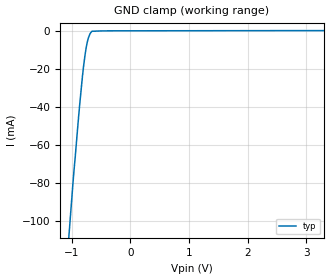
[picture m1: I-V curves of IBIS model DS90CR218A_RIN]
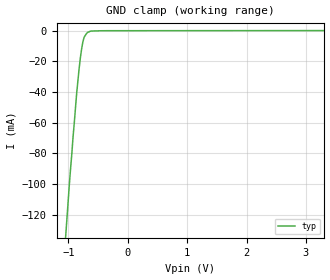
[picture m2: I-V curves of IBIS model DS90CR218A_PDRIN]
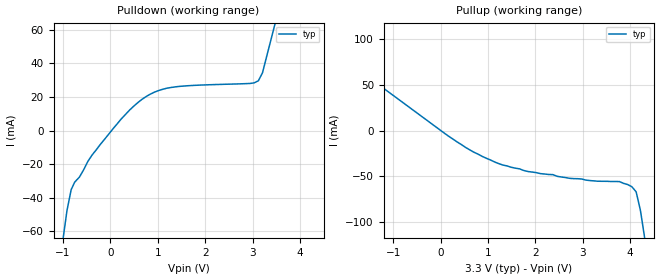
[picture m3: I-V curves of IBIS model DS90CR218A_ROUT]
|   National Semiconductor Corporation
|   Interface Products Group
|   IBIS Model of DS90CR218AMTD
|   High Speed Link Receiver
|   48L TSSOP
[IBIS Ver]   2.1
[Comment char]  |_char
[File name]   90cr218a.ibs
[File Rev]   1.3
[Date]   7/27/00
[Source]   File originated at National Semiconductor Corporation.
   Interface Group/Analog Division. All data based on
   Empirical Measurements(Bench).
[Notes]   File created by DT.
   Revision 1.0: The original model.
   Revision 1.1: Corrected driver output pulldown
   and pullup.
   Revision 1.2: Corrected ground and power clamp data.
   Revision 1.3: Changed Vih/Vil of LVDS Input to 100mV
   Deleted V/T data because it was wrong.
[Disclaimer]
(C) Copyright National Semiconductor Corporation 2000
   All rights reserved
   National Semiconductor Corporation hereby grants
the user of this IBIS model a non-exclusive, nontransferable
license to use this IBIS model under the following terms.
Before using this IBIS model, the user should read this
license.  If the user does not accept these terms, the
IBIS model should be returned to National within 30 days.
   The user is granted this license only to use the
IBIS model and is not granted rights to sell, load, rent,
lease or license the IBIS model in whole or in part, or in
modified form to anyone other than user. User may modify
the IBIS model to suit its specific applications but rights
to derivative works and such modifications shall belong to
National.
   This IBIS model is provided on an "AS IS" basis and
National makes absolutely no warranty with respect to the
information contained herein. NATIONAL DISCLAIMS AND CUSTOMER
WAIVES ALL WARRANTIES, EXPRESS OR IMPLIED, INCLUDING
WARRANTIES OF MERCHANTABILITY OR FITNESS FOR A PARTICULAR
PURPOSE. The entire risk as to quality and performance is
with the Customer. ACCORDINGLY, IN NO EVENT SHALL THE
COMPANY BE LIABLE FOR ANY DAMAGES, WHETHER IN CONTRACT OR
TORT,INCLUDING ANY LOST PROFITS OR OTHER INCIDENTAL,
CONSEQUENTIAL, EXEMPLARY, OR PUNITIVE DAMAGES ARISING OUT
OF THE USE OR APPLICATION OF THE IBIS model provided in
this package. Further, National reserves the right to make
changes without notice to any product herein to improve
reliability, function, or design. National does not convey
any license under patent rights or any other intellectual
property rights, including those of third parties.
   National is not obligated to provide maintenance or support
for the licensed IBIS model.
Contact National at ATTN:INTERFACE APPLICATIONS/IBIS MODELS.
2900 Semiconductor Drive, M/S A2595, Santa Clara, CA 95052-8090
[Copyright]   Copyright 2000, National Semiconductor, All Rights Reserved
[Component]   DS90CR218AMTD
[Manufacturer]  National Semiconductor Corp
[Package]
|   typ   min   max
R_pkg   97.97m   NA   NA
L_pkg   3.000nH   NA   NA
C_pkg   0.2108pF   NA   NA
[Pin]   signal_name   model_name   R_pin   L_pin   C_pin
1   RxOUT17   DS90CR218A_ROUT   68.8m  2.270n  0.3587p
2   RxOUT18   DS90CR218A_ROUT   65.4m  2.200n  0.3414p
3   GND   GND   133.7m  3.880n  0.3183p
4   RxOUT19   DS90CR218A_ROUT   121.7m  3.590n  0.2610p
5   RxOUT20   DS90CR218A_ROUT   120.6m  3.510n  0.2205p
6   N/C   NC   117.6m  3.460n  0.1689p
7   LVDSGND   GND   104.9m  3.170n  0.1594p
8   RxIN0-   DS90CR218A_RIN   97.8m  2.970n  0.1515p
9   RxIN0+   DS90CR218A_RIN   92.6m  2.860n  0.1459p
10   RxIN1-   DS90CR218A_RIN   92.6m  2.840n  0.1459p
11   RxIN1+   DS90CR218A_RIN   94.0m  2.800n  0.1568p
12   LVDSVCC   POWER   81.7m  2.640n  0.1311p
13   LVDSGND   GND   73.9m  2.660n  0.1116p
14   RxIN2-   DS90CR218A_RIN   89.6m  2.720n  0.1343p
15   RxIN2+   DS90CR218A_RIN   87.2m  2.860n  0.1384p
16   RxCLKIN-   DS90CR218A_RIN   92.6m  2.880n  0.1458p
17   RxCLKIN+   DS90CR218A_RIN   98.8m  3.040n  0.1563p
18   LVDSGND   GND   102.9m  3.160n  0.1572p
19   PLLGND   GND   111.4m  3.210n  0.1639p
20   PLLVCC   POWER   113.5m  3.340n  0.2126p
21   PLLGND   GND   121.8m  3.590n  0.2606p
22   PWRDWN*   DS90CR218A_PDRIN   133.8m  3.880n  0.3183p
23   RxCLKOUT   DS90CR218A_ROUT   65.5m  2.200n  0.3414p
24   RxOUT0   DS90CR218A_ROUT   68.8m  2.270n  0.3587p
25   GND   GND   68.8m  2.270n  0.3587p
26   RxOUT1   DS90CR218A_ROUT   65.5m  2.200n  0.3414p
27   RxOUT2   DS90CR218A_ROUT   133.8m  3.880n  0.3183p
28   VCC   POWER   121.8m  3.590n  0.2606p
29   RxOUT3   DS90CR218A_ROUT   113.5m  3.340n  0.2126p
30   RxOUT4   DS90CR218A_ROUT   111.4m  3.210n  0.1639p
31   RxOUT5   DS90CR218A_ROUT   102.9m  3.160n  0.1572p
32   GND   GND   98.8m  3.040n  0.1563p
33   RxOUT6   DS90CR218A_ROUT   92.6m  2.880n  0.1458p
34   RxOUT7   DS90CR218A_ROUT   87.2m  2.860n  0.1384p
35   RxOUT8   DS90CR218A_ROUT   89.6m  2.720n  0.1343p
36   VCC   POWER   73.9m  2.660n  0.1116p
37   RxOUT9   DS90CR218A_ROUT   81.7m  2.640n  0.1311p
38   GND   GND   94.0m  2.800n  0.1568p
39   RxOUT10   DS90CR218A_ROUT   92.6m  2.840n  0.1459p
40   RxOUT11   DS90CR218A_ROUT   92.6m  2.860n  0.1459p
41   RxOUT12   DS90CR218A_ROUT   97.8m  2.970n  0.1515p
42   VCC   POWER   104.9m  3.170n  0.1594p
43   RxOUT13   DS90CR218A_ROUT   117.6m  3.460n  0.1689p
44   GND   GND   120.6m  3.510n  0.2205p
45   RxOUT14   DS90CR218A_ROUT   121.7m  3.590n  0.2610p
46   RxOUT15   DS90CR218A_ROUT   133.7m  3.880n  0.3183p
47   RxOUT16   DS90CR218A_ROUT   65.4m  2.200n  0.3414p
48   VCC   POWER   68.8m  2.270n  0.3587p
[Diff_pin]   inv_pin   vdiff   tdelay_typ   tdelay_min   tdelay_max
| The '+' pin is Diff_pin and the '-' pin is the inv_pin
9   8   0.1   0   0   0
11   10   0.1   0   0   0
15   14   0.1   0   0   0
17   16   0.1   0   0   0
| Models and submodels in the file (3): DS90CR218A_RIN (Input), DS90CR218A_PDRIN (Input), DS90CR218A_ROUT (3-state)
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|   RECEIVER INPUT  MODEL
[Model]   DS90CR218A_RIN
Model_type   Input
|Signals   RxIN+,RxIN- ; RxCLKIN+, RxCLKIN-
Vinh = .1
Vinl = -.1
|   typ   min   max
C_comp   5.247pF   NA   NA
|   typ   min   max
[Temperature Range]   25.0   NA   NA
[Voltage range]   3.3V   3.0V   3.6V
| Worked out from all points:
|   GND clamp passes 1 mA (typ) near -0.68 V on its own axis
[Power_clamp]
| Note that the[POWER_clamp]voltage table is referenced to Vcc
| and is calculated using Vtable=Vcc - Vmeasured.
|Voltage   I(typ)   I(min)   I(max)
-3V       0A         NA         NA
0V        0A         NA         NA
[GND_clamp]
|Voltage   I(typ)   I(min)   I(max)
-3.3V     -1.012A    NA         NA
-1.002V   -88.22mA   NA         NA
-962.8mV  -73.12mA   NA         NA
-941.2mV  -65.81mA   NA         NA
-880.7mV  -43.69mA   NA         NA
-818.7mV  -23.78mA   NA         NA
-798.1mV  -18.11mA   NA         NA
-756.8mV  -9.025mA   NA         NA
-735.6mV  -5.759mA   NA         NA
-691.4mV  -1.641mA   NA         NA
-655mV    -228.3uA   NA         NA
3.3V      116.3uA    NA         NA
|   RECEIVER PWRDWN* INPUT MODEL
[Model]   DS90CR218A_PDRIN
Model_type   Input
|Signals   PWRDWN*
Vinh = 2.0
Vinl = 0.8
|   typ   min   max
C_comp   5.400pF   NA   NA
|   typ   min   max
[Temperature Range]   25.0   NA   NA
[Voltage range]   3.3V   3.0V   3.6V
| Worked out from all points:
|   GND clamp passes 1 mA (typ) near -0.67 V on its own axis
[GND_clamp]
|Voltage   I(typ)   I(min)   I(max)
-3.3V     -1.368A    NA         NA
-1.002V   -110.2mA   NA         NA
-984mV    -100.2mA   NA         NA
-923mV    -69.93mA   NA         NA
-861mV    -40.95mA   NA         NA
-818.7mV  -24.46mA   NA         NA
-798.1mV  -17.54mA   NA         NA
-757.3mV  -7.457mA   NA         NA
-736.1mV  -4.382mA   NA         NA
-672.4mV  -944.6uA   NA         NA
-449.4mV  -31.18uA   NA         NA
3.3V      84.23uA    NA         NA
[Power_clamp]
| Note that the[POWER_clamp]voltage table is referenced to Vcc
| and is calculated using Vtable=Vcc - Vmeasured.
|Voltage   I(typ)   I(min)   I(max)
-3.3V     0A         0A         0A
0V        0A         0A         0A
|   RECEIVER OUTPUT  MODEL
[Model]   DS90CR218A_ROUT
Model_type   3-state
| Signals   RxOUT0 ~ RxOUT20
Vmeas = 1.5V   |This is 0.0v differential on output
Cref = 8pF   |Timing specification test load capacitance value
Vref = 0   |Timing specification test load voltage; GND
| variable   typ   min   max
C_comp   3.720pF   NA   NA
|   typ   min   max
[Temperature Range]   25.0   NA   NA
[Voltage range]   3.3V   3.0V   3.6V
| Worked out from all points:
|   slope of the pulldown table from 0 to 0.495 V, typ, clamps not added: 32 ohm
|   slope of the pullup table from 0 to 0.495 V, typ, clamps not added: 28.4 ohm
[Pulldown]
| Voltage   I(typ)   I(min)   I(max)
-3.3V     -535.4mA   NA         NA
-1.002V   -65.19mA   NA         NA
-827.6mV  -35.25mA   NA         NA
-475mV    -18.38mA   NA         NA
402.7mV   12.11mA    NA         NA
929.9mV   22.88mA    NA         NA
1.456V    26.3mA     NA         NA
3.036V    28.41mA    NA         NA
3.124V    29.65mA    NA         NA
3.211V    34.39mA    NA         NA
3.299V    44.1mA     NA         NA
6.6V      408mA      NA         NA
[Pullup]
| Note that the[Pullup]voltage table is referenced to Vcc
| and is calculated using Vtable=Vcc - Vmeasured.
|Voltage   I(typ)   I(min)   I(max)
-3.3V     126mA      NA         NA
351.7mV   -12.52mA   NA         NA
877.5mV   -28.16mA   NA         NA
1.317V    -37.67mA   NA         NA
1.849V    -44.74mA   NA         NA
3.159V    -54.6mA    NA         NA
3.775V    -55.67mA   NA         NA
4.038V    -61.28mA   NA         NA
4.128V    -66.85mA   NA         NA
4.219V    -87.07mA   NA         NA
4.301V    -114.7mA   NA         NA
6.6V      -887.3mA   NA         NA
[GND_clamp]
| Outputs in Tri-state.
| Voltage   I(typ)   I(min)   I(max)
| Receiver output is non-tristable
-3V       0A         NA         NA
3V        0A         NA         NA
[POWER_clamp]
| Note that the[POWER_clamp]voltage table is referenced to Vcc
| and is calculated using Vtable=Vcc - Vmeasured.
| Outputs in Tri-state.
|Voltage   I(typ)   I(min)   I(max)
| Receiver output is non-tristable
-3V       0A         NA         NA
0V        0A         NA         NA
[Ramp]
| Note: Ramp rate measured on single-ended Driver Output.
|   typ   min   max
dV/dt_r   1.962/1.0754n   NA   NA
dV/dt_f   1.950/1.0088n   NA   NA
R_load = 1MOhm  | Represent Hi-Z
